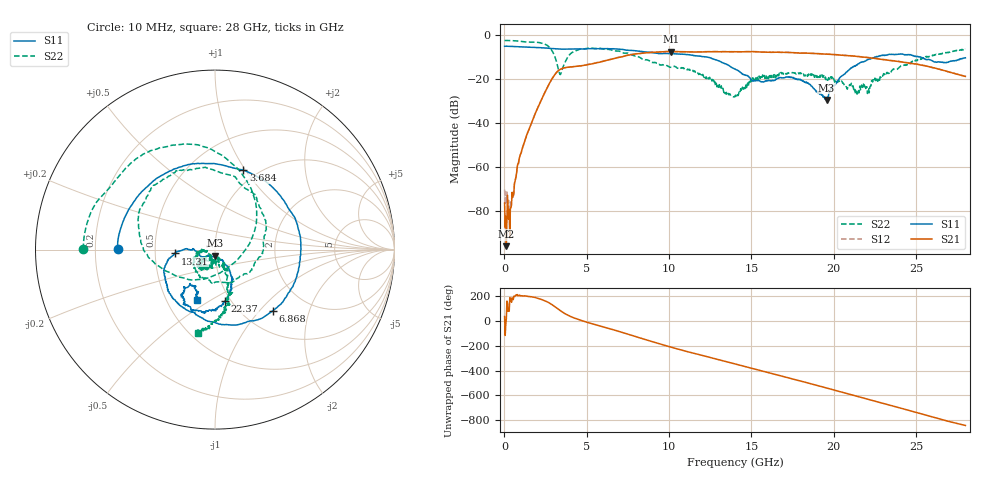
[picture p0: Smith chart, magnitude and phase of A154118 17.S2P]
!  2-Port S-parameters saved by WinCal
! VAR MeasName=S-Parameters (CALIBRATED_DATA) read from VNA (N5230A)
! VAR MeasDate=2015-9-10 14:35:42
! VAR NAME=A154118 17
! VAR FILENAME=A154118 17.S2P
! VAR DATE=2015-9-10 14:35:42
! VAR PHYS_PORTS=1,2
# Hz S DB R 50
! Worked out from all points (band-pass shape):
!   801 points, 10 MHz to 28 GHz, reference 50 ohm
!   highest |S21| = -7.70 dB at 10.12 GHz (marker M1); lowest = -96.0 dB at 115 MHz (marker M2)
!   |S21| within 3 dB of the highest: 6.75 GHz to 22.34 GHz (15.59 GHz wide, 107 % of centre)
!   lowest |S11| = -29.6 dB at 19.57 GHz (marker M3), VSWR 1.07, Z = 50.1 - j3.31 ohm
!   |S11| at or under -10 dB: 12.12 GHz to 22.6 GHz (10.48 GHz wide, 60.3 % of centre); 25.0922 GHz to 25.15601 GHz (63.8 MHz wide, 0.254 % of centre); 25.17 GHz to end of sweep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
!   |S22| runs from -28.5 to -2.7 dB; largest |S21 - S12| = 0.0076
!   S11 on the Smith chart (normalised r, x): 10 MHz: 0.30, +0.00; 3.684 GHz: 0.86, +0.98; 6.868 GHz: 1.35, -1.18; 13.31 GHz: 0.64, -0.03; 22.37 GHz: 0.94, -0.59; 28 GHz: 0.71, -0.43
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1e7  -5.32 179.6  -76.40 33.5  -70.37 154.2  -2.67 179.8
1.149625e8  -5.29 176.5  -96.01 15.5  -76.29 67.2  -2.69 177.2
4.2985e8  -5.38 167.0  -77.26 148.3  -74.75 159.9  -2.75 169.5
1.024638e9  -5.60 150.4  -53.41 -159.6  -53.45 -160.5  -3.12 154.9
2.459125e9  -6.08 108.6  -26.20 159.8  -26.17 160.1  -4.38 103.6
3.0889e9  -6.43 88.7  -17.87 110.9  -17.87 111.0  -10.58 38.2
3.3688e9  -6.60 80.5  -15.87 83.5  -15.87 83.4  -18.09 -43.9
3.683688e9  -6.57 70.3  -15.02 56.3  -15.03 56.5  -12.54 -138.1
4.698325e9  -6.56 33.6  -14.13 0.9  -14.12 1.0  -6.49 152.5
6.86755e9  -6.58 -46.7  -10.50 -82.6  -10.40 -82.8  -7.46 76.9
9.351662e9  -8.60 -107.5  -7.95 177.7  -7.89 177.2  -13.52 -40.0
1.012139e10  -8.63 -118.4  -7.70 147.5  -7.67 147.0  -14.86 -86.1
1.330525e10  -13.00 -174.5  -7.75 37.1  -7.73 36.5  -25.63 -164.4
1.4005e10  -15.68 178.3  -7.79 13.2  -7.77 12.6  -27.94 -132.8
1.51246e10  -21.10 -170.5  -7.75 -25.6  -7.76 -26.3  -20.69 -100.5
1.662906e10  -19.91 -135.7  -8.01 -76.7  -7.97 -77.3  -18.73 -120.8
1.869332e10  -23.57 -140.6  -8.54 -149.2  -8.54 -149.6  -18.00 -131.5
1.956801e10  -29.62 -86.9  -8.88 179.6  -8.80 179.0  -20.35 -145.2
2.138736e10  -13.76 -62.0  -9.89 113.9  -9.78 113.2  -25.68 -117.5
2.236701e10  -10.66 -79.3  -10.72 78.8  -10.65 77.7  -21.51 -76.4
2.334666e10  -9.05 -98.4  -11.69 43.6  -11.56 42.6  -17.47 -58.4
2.8e10  -10.54 -110.1  -18.98 -121.3  -19.01 -122.3  -6.44 -101.3
